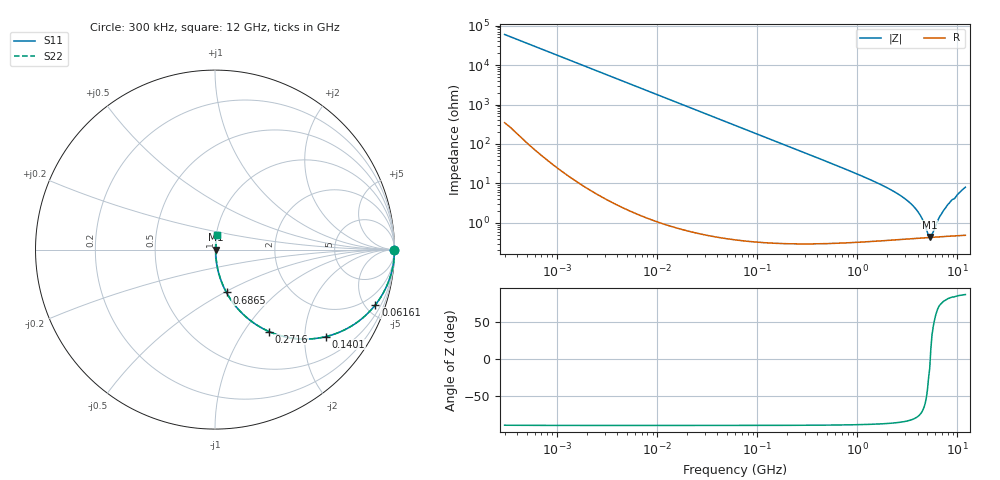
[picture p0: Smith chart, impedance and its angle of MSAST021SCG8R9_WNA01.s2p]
! MSAST021SCG8R9_WNA01  S-PARAMETER MODEL  ( General Type )
! Model Generated by TAIYO YUDEN Corporation (http://www.ty-top.com)
! Version 2.0
! TAIYO YUDEN Control No. 181101
! Copyright(c) 2015 TAIYO YUDEN CO.,LTD. All Rights Reserved.
! Product Description (link to TY-COMPAS)
! https://ds.yuden.co.jp/TYCOMPAS/or/detail?pn=MSAST021SCG8R9CWNA01&u=M
! Products Name : Multilayer Ceramic Capacitors
! Characteristics :
!  Capacitance : 8.9 pF , Rated Voltage : 25V , TCC : CG / C0G
!  Case Size : 0.25 x 0.125 / 0.0098 x 0.0049 [mm/inch] , Thickness : 0.125 / 0.0049 [mm/inch]
!  (Conditions: Temperature = 25 degC , DC Bias Current/Voltage = 0A / 0V)
! External Node Assignments :
!  1  o---| |---o  2
! GND o---------o GND
! Frequency Range : 0.3MHz  -  12000MHz  [ 401 STEP ]
# MHz S RI R 50
! Freq[MHz].  S11 Real  S11 Imag  S21 Real  S21 Imag  S12 Real  S12 Imag  S22 Real  S22 Imag
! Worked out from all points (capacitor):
!   401 points, 300 kHz to 12 GHz, reference 50 ohm
!   read as one part in series: C = 8.9 pF near 316.3 kHz
!   lowest |Z| = 439 mohm at 5.279 GHz (marker M1)
!   series resonance near 5.35 GHz, so ESL is about 99 pH
!   S11 on the Smith chart (normalised r, x): 300 kHz: open; 61.61 MHz: 1.01, -5.80; 140.1 MHz: 1.01, -2.55; 271.6 MHz: 1.01, -1.31; 686.5 MHz: 1.01, -0.51; 12 GHz: 1.01, +0.16
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0.3  1 -0.00168  1.26e-05 0.00168  1.26e-05 0.00168  1 -0.00168
1.769972  0.9999 -0.0099  0.000107 0.0099  0.000107 0.0099  0.9999 -0.0099
10.44266  0.9966 -0.0582  0.00343 0.0582  0.00343 0.0582  0.9966 -0.0582
26.39317  0.9786 -0.1444  0.0214 0.1444  0.0214 0.1444  0.9786 -0.1444
60  0.8985 -0.3014  0.1015 0.3014  0.1015 0.3014  0.8985 -0.3014
61.61074  0.8936 -0.3078  0.1064 0.3078  0.1064 0.3078  0.8936 -0.3078
91.67136  0.7914 -0.4055  0.2086 0.4055  0.2086 0.4055  0.7914 -0.4055
140.0606  0.6192 -0.4844  0.3808 0.4844  0.3808 0.4844  0.6192 -0.4844
271.6094  0.3021 -0.4569  0.6979 0.4569  0.6979 0.4569  0.3021 -0.4569
353.9943  0.2033 -0.3995  0.7967 0.3995  0.7967 0.3995  0.2033 -0.3995
686.4755  0.0641 -0.239  0.9359 0.239  0.9359 0.239  0.0641 -0.239
2088.533  0.00876 -0.0715  0.9912 0.0715  0.9912 0.0715  0.00876 -0.0715
2947.191  0.00557 -0.0416  0.9944 0.0416  0.9944 0.0416  0.00557 -0.0416
3740.715  0.00457 -0.0238  0.9954 0.0238  0.9954 0.0238  0.00457 -0.0238
4385.161  0.00428 -0.0128  0.9957 0.0128  0.9957 0.0128  0.00428 -0.0128
5006.236  0.00423 -0.00387  0.9958 0.00387  0.9958 0.00387  0.00423 -0.00387
5278.635  0.00425 -0.00101  0.9957 0.00101  0.9957 0.00101  0.00425 -0.00101
5565.855  0.00429 0.00265  0.9957 -0.00265  0.9957 -0.00265  0.00429 0.00265
6699.894  0.00462 0.0141  0.9954 -0.0141  0.9954 -0.0141  0.00462 0.0141
7648.807  0.00509 0.0238  0.9949 -0.0238  0.9949 -0.0238  0.00509 0.0238
10511.28  0.00814 0.0581  0.9919 -0.0581  0.9919 -0.0581  0.00814 0.0581
12000  0.0111 0.0787  0.9889 -0.0787  0.9889 -0.0787  0.0111 0.0787
